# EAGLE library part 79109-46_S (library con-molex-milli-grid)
RECEPTACAL
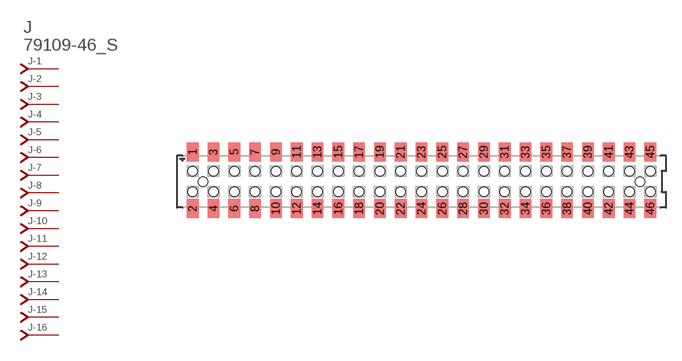
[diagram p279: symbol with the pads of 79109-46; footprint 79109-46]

Designator prefix J; gates -1=J-NV -2=J-N -3=J-N -4=J-N -5=J-N -6=J-N -7=J-N -8=J-N -9=J-N -10=J-N -11=J-N -12=J-N -13=J-N -14=J-N -15=J-N -16=J-N -17=J-N -18=J-N -19=J-N -20=J-N -21=J-N -22=J-N -23=J-N -24=J-N -25=J-N -26=J-N -27=J-N -28=J-N -29=J-N -30=J-N -31=J-N -32=J-N -33=J-N -34=J-N -35=J-N -36=J-N -37=J-N -38=J-N -39=J-N -40=J-N -41=J-N -42=J-N -43=J-N -44=J-N -45=J-N -46=J-N

## 79109-46_S  [79109-46]
1  -1:J  pas
2  -2:J  pas
3  -3:J  pas
4  -4:J  pas
5  -5:J  pas
6  -6:J  pas
7  -7:J  pas
8  -8:J  pas
9  -9:J  pas
10  -10:J  pas
11  -11:J  pas
12  -12:J  pas
13  -13:J  pas
14  -14:J  pas
15  -15:J  pas
16  -16:J  pas
17  -17:J  pas
18  -18:J  pas
19  -19:J  pas
20  -20:J  pas
21  -21:J  pas
22  -22:J  pas
23  -23:J  pas
24  -24:J  pas
25  -25:J  pas
26  -26:J  pas
27  -27:J  pas
28  -28:J  pas
29  -29:J  pas
30  -30:J  pas
31  -31:J  pas
32  -32:J  pas
33  -33:J  pas
34  -34:J  pas
35  -35:J  pas
36  -36:J  pas
37  -37:J  pas
38  -38:J  pas
39  -39:J  pas
40  -40:J  pas
41  -41:J  pas
42  -42:J  pas
43  -43:J  pas
44  -44:J  pas
45  -45:J  pas
46  -46:J  pas

## Footprint 79109-46 (pad centres in mm)
RECEPTACAL SMD Dual Row, Vertical, Pass-Thru
smd 1.12 x 1.83: 1 -22,2.85; 2 -22,-2.6; 3 -20,2.85; 4 -20,-2.6; 5 -18,2.85; 6 -18,-2.6; 7 -16,2.85; 8 -16,-2.6; 9 -14,2.85; 10 -14,-2.6; 11 -12,2.85; 12 -12,-2.6; 13 -10,2.85; 14 -10,-2.6; 15 -8,2.85; 16 -8,-2.6; 17 -6,2.85; 18 -6,-2.6; 19 -4,2.85; 20 -4,-2.6; 21 -2,2.85; 22 -2,-2.6; 23 0,2.85; 24 0,-2.6; 25 2,2.85; 26 2,-2.6; 27 4,2.85; 28 4,-2.6; 29 6,2.85; 30 6,-2.6; 31 8,2.85; 32 8,-2.6; 33 10,2.85; 34 10,-2.6; 35 12,2.85; 36 12,-2.6; 37 14,2.85; 38 14,-2.6; 39 16,2.85; 40 16,-2.6; 41 18,2.85; 42 18,-2.6; 43 20,2.85; 44 20,-2.6; 45 22,2.85; 46 22,-2.6
hole 0.914 at -21,0
hole 0.914 at -22,1
hole 0.914 at -22,-1
hole 0.914 at -20,-1
hole 0.914 at -20,1
hole 0.914 at -18,-1
hole 0.914 at -18,1
hole 0.914 at -16,1
hole 0.914 at -16,-1
hole 0.914 at -14,1
hole 0.914 at -14,-1
hole 0.914 at -12,1
hole 0.914 at -12,-1
hole 0.914 at -10,1
hole 0.914 at -10,-1
hole 0.914 at -8,-1
hole 0.914 at -8,1
hole 0.914 at -6,1
hole 0.914 at -6,-1
hole 0.914 at -4,1
hole 0.914 at -4,-1
hole 0.914 at -2,1
hole 0.914 at -2,-1
hole 0.914 at 0,-1
hole 0.914 at 0,1
hole 0.914 at 2,1
hole 0.914 at 4,1
hole 0.914 at 6,1
hole 0.914 at 2,-1
hole 0.914 at 4,-1
hole 0.914 at 6,-1
hole 0.914 at 8,-1
hole 0.914 at 10,-1
hole 0.914 at 12,-1
hole 0.914 at 14,-1
hole 0.914 at 16,-1
hole 0.914 at 8,1
hole 0.914 at 10,1
hole 0.914 at 12,1
hole 0.914 at 14,1
hole 0.914 at 16,1
hole 0.914 at 18,-1
hole 0.914 at 20,-1
hole 0.914 at 18,1
hole 0.914 at 20,1
hole 0.914 at 22,1
hole 0.914 at 22,-1
hole 0.914 at 21,0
